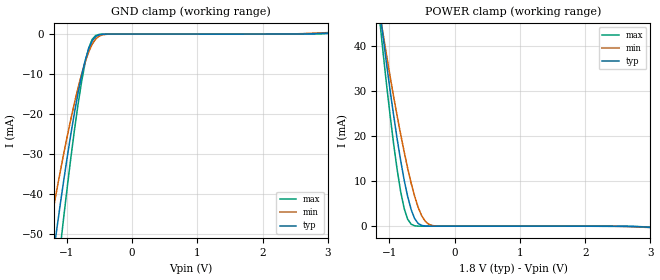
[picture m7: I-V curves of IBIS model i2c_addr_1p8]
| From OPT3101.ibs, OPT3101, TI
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|   i2c_addr_1p8 Model
[Model]   i2c_addr_1p8
Model_type   Input
Vinl = 0.54
Vinh = 1.26
|   typ   min   max
|   (nom PVT)   (fast PVT)   (slow PVT)
C_comp   2.094e-12   1.903e-12   2.287e-12
[Model spec]
|subparameter
Vinl   0.54   0.51   0.57
Vinh   1.26   1.19   1.33
| Where nom  PVT is Nominal Process, 1.8V, 27C
|   Fast PVT is Strong Process,  1.9V, -40C
|   Slow PVT is Weak Process,   1.7V, 125C
[Voltage Range]   1.8   1.7   1.9
|Junction Temperature
[Temperature Range]   27   125   -40
[Power Clamp Reference]   1.8   1.7   1.9
[GND Clamp Reference]   0   0   0
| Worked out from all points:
|   GND clamp passes 1 mA (typ) near -0.58 V on its own axis
|   POWER clamp passes 1 mA (typ) near -0.58 V on its own axis
[GND Clamp]
|   Voltage   I(typ)   I(min)   I(max)
-1.8V     -227.8mA   -113.9mA   -384.9mA
-1.26V    -61.63mA   -48.52mA   -77.43mA
-1.152V   -48.54mA   -38.8mA    -60.98mA
-1.098V   -42.25mA   -34.12mA   -53.01mA
-1.044V   -36.16mA   -29.6mA    -45.25mA
-882mV    -19.52mA   -17.11mA   -23.79mA
-774mV    -10.34mA   -10.02mA   -11.89mA
-666mV    -3.676mA   -4.479mA   -3.522mA
-612mV    -1.672mA   -2.525mA   -1.315mA
-558mV    -595.6uA   -1.216mA   -357.1uA
-342mV    -1.956uA   -16.22uA   -918.5nA
3.6V      749.5uA    779.3uA    763.2uA
[POWER Clamp]
|   Voltage   I(typ)   I(min)   I(max)
-1.8V     228mA      188mA      226mA
-1.152V   48.5mA     47.8mA     46.4mA
-1.098V   42.3mA     42.9mA     38.8mA
-936mV    24.8mA     28.9mA     18.4mA
-828mV    14.7mA     20.5mA     7.77mA
-774mV    10.3mA     16.6mA     3.97mA
-720mV    6.62mA     12.9mA     1.55mA
-666mV    3.68mA     9.55mA     441uA
-612mV    1.67mA     6.61mA     95.2uA
-504mV    169uA      2.29mA     2.76uA
-342mV    1.96uA     147uA      773nA
3.6V      -750uA     -710uA     -870uA
